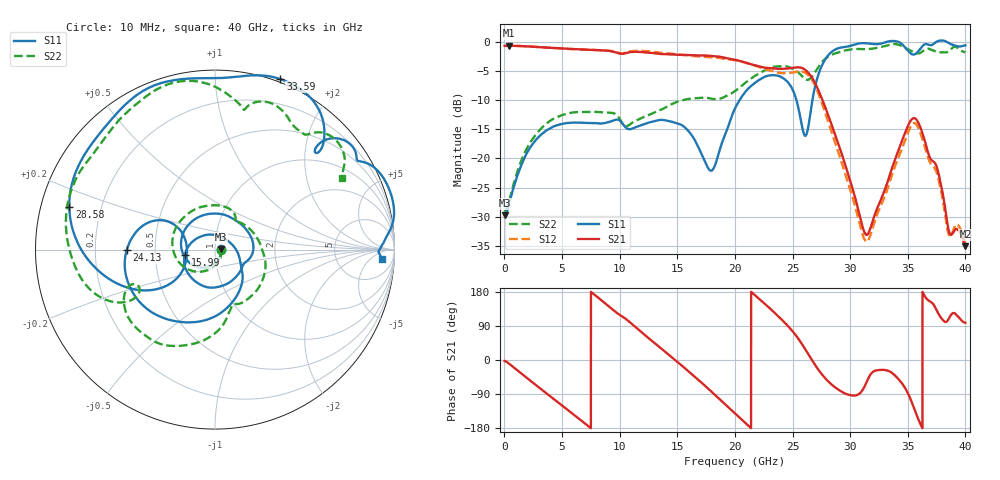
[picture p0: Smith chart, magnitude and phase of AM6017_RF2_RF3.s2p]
!Agilent Technologies,E8364B,MY43040894,A.07.50.67
!Agilent E8364B: A.07.50.67
!Date: Wednesday, July 17, 2019 10:35:59
!Correction: S11(Full 2 Port(1,2))
!S21(Full 2 Port(1,2))
!S12(Full 2 Port(1,2))
!S22(Full 2 Port(1,2))
!S2P File: Measurements: S11, S21, S12, S22:
# Hz S  dB  R 50
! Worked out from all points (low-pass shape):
!   6401 points, 10 MHz to 40 GHz, reference 50 ohm
!   highest |S21| = -0.65 dB at 409.9 MHz (marker M1); lowest = -35.1 dB at 40 GHz (marker M2)
!   |S21| within 3 dB of the highest: start of sweep to 21.06 GHz
!   lowest |S11| = -29.8 dB at 10 MHz (marker M3), VSWR 1.07, Z = 53.3 + j0.235 ohm
!   |S11| at or under -10 dB: start of sweep to 20.4 GHz; 25.34 GHz to 26.72 GHz (1.387 GHz wide, 5.33 % of centre)
!   |S22| runs from -29.2 to -0.4 dB; largest |S21 - S12| = 0.058
!   S11 on the Smith chart (normalised r, x): 10 MHz: 1.07, +0.00; 15.99 GHz: 0.71, -0.04; 24.13 GHz: 0.34, -0.00; 28.58 GHz: 0.09, +0.14; 33.59 GHz: -0.03, +1.45; 40 GHz: 17, -14
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1e7  -29.77 3.9  -0.67 -2.4  -0.74 -1.9  -29.23 -7.0
4.099e8  -27.76 -37.0  -0.65 -10.0  -0.65 -10.0  -27.26 -36.8
3.502877e9  -15.40 -162.0  -0.97 -84.7  -0.98 -84.7  -14.25 -148.6
6.677083e9  -13.86 111.6  -1.29 -160.2  -1.31 -160.0  -12.03 141.5
8.520372e9  -14.01 54.7  -1.47 155.0  -1.46 155.5  -12.12 100.1
1.082605e10  -14.99 -27.9  -1.78 101.2  -1.67 101.5  -14.24 53.1
1.334417e10  -13.45 -93.6  -2.02 36.4  -1.81 35.1  -11.84 5.4
1.598725e10  -15.37 -169.9  -2.27 -30.3  -2.35 -32.8  -9.79 -42.8
1.798051e10  -22.10 62.8  -2.41 -83.9  -2.66 -85.4  -9.77 -69.3
2.0005e10  -11.43 -59.8  -3.07 -141.0  -3.16 -142.0  -8.45 -79.4
2.197326e10  -6.70 -121.4  -4.14 164.5  -4.23 161.3  -5.55 -100.8
2.412897e10  -6.16 -179.6  -4.63 104.5  -5.38 101.3  -4.17 -135.0
2.605974e10  -16.08 176.7  -4.74 30.4  -5.26 29.8  -6.33 -156.4
2.667208e10  -10.62 -142.6  -6.09 0.5  -6.46 -1.6  -6.00 -149.4
2.857786e10  -1.46 163.7  -15.25 -69.5  -16.57 -72.5  -2.07 -173.9
3.135216e10  -0.24 105.0  -33.04 -63.2  -34.24 -58.0  -1.28 142.3
3.333917e10  0.09 73.4  -23.48 -29.0  -24.62 -23.8  -0.56 113.9
3.35891e10  0.15 69.0  -21.93 -33.2  -23.06 -27.7  -0.43 109.3
3.571982e10  -2.01 45.2  -13.26 -141.2  -14.10 -132.2  -1.93 78.8
3.757561e10  0.10 25.2  -21.86 126.9  -22.85 138.1  -1.75 57.9
3.856911e10  -0.23 5.7  -32.49 109.7  -33.15 129.0  -1.62 50.9
4e10  -0.59 -3.3  -35.06 98.3  -34.61 106.6  -1.80 29.4
